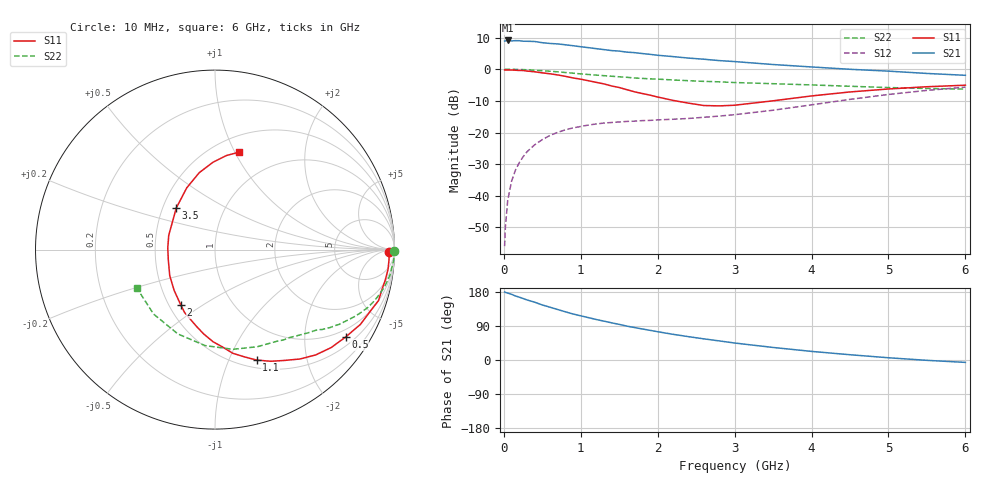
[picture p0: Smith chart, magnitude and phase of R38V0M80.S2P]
! SIEMENS Small Signal Semiconductors
! BFR181
! Si NPN RF Bipolar Junction Transistor in SOT23
! VCE = 8 V  IC = 0.8 mA
! Common Emitter S-Parameters:  May  1996
# GHz  S  MA  R  50
!  f  S11  S21  S12  S22
! GHz  MAG  ANG  MAG  ANG  MAG  ANG  MAG  ANG
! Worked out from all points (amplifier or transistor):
!   36 points, 10 MHz to 6 GHz, reference 50 ohm
!   highest |S21| = 9.1 dB at 50 MHz (marker M1)
!   |S21| within 3 dB of that: start of sweep to 1.337 GHz
!   unconditionally stable (mu >= 1): 2.182 GHz to 3.789 GHz
!   at 250 MHz: K = 0.14, MSG = 18.3 dB, |S12| = -27.7 dB
!   at 1.4 GHz: K = 0.70, MSG = 11.4 dB, |S12| = -16.8 dB
!   at 6 GHz: K = 0.88, MSG = 1.9 dB, |S12| = -5.7 dB
!   S11 on the Smith chart (normalised r, x): 10 MHz: 60, -26; 500 MHz: 0.75, -3.13; 1.1 GHz: 0.59, -1.27; 2 GHz: 0.57, -0.41; 3.5 GHz: 0.59, +0.30; 6 GHz: 0.66, +1.04
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0.01  0.9722 -0.7  2.785 179.5  0.0016 90.4  0.9983 -0.3
0.02  0.9705 -1.5  2.797 178.3  0.0032 89.6  0.9916 -0.7
0.05  0.9712 -3.6  2.846 176.6  0.0084 88.8  0.9985 -1.7
0.1  0.9701 -6.7  2.798 173.4  0.0169 86.3  0.9976 -3.3
0.15  0.9634 -10.3  2.828 169.0  0.0253 82.7  0.9919 -5.0
0.2  0.956 -13.7  2.82 165.8  0.0333 80.8  0.9882 -6.5
0.4  0.9107 -27.3  2.742 152.6  0.0638 72.1  0.9648 -12.8
0.5  0.8756 -33.8  2.623 145.2  0.0772 68.1  0.9463 -15.7
0.7  0.8119 -46.3  2.509 133.2  0.1005 60.8  0.9086 -20.9
0.8  0.7715 -52.2  2.43 127.2  0.1103 57.2  0.8869 -23.2
0.9  0.7276 -58.1  2.351 121.4  0.1183 54.4  0.865 -25.4
1.1  0.6574 -69.4  2.191 111.8  0.1312 49.7  0.8251 -29.2
1.4  0.5441 -85.6  1.969 98.1  0.1439 44.5  0.7746 -34.1
1.6  0.4745 -97.6  1.861 89.4  0.1497 42.3  0.745 -36.7
2  0.3635 -121.5  1.66 74.6  0.1584 41.4  0.6971 -41.6
2.2  0.3213 -135.2  1.582 67.8  0.1619 42.0  0.6761 -44.4
2.6  0.2668 -167.0  1.438 55.8  0.174 44.6  0.6423 -49.7
3  0.2697 162.9  1.32 44.8  0.1912 47.6  0.6157 -56.1
3.5  0.3168 132.9  1.186 33.1  0.2249 50.3  0.5902 -66.5
4.5  0.4373 101.6  0.997 13.9  0.3338 48.3  0.5376 -95.9
5.5  0.5284 83.0  0.857 -0.9  0.4627 36.4  0.4961 -133.6
6  0.559 76.1  0.801 -6.3  0.5208 28.4  0.4851 -153.7
